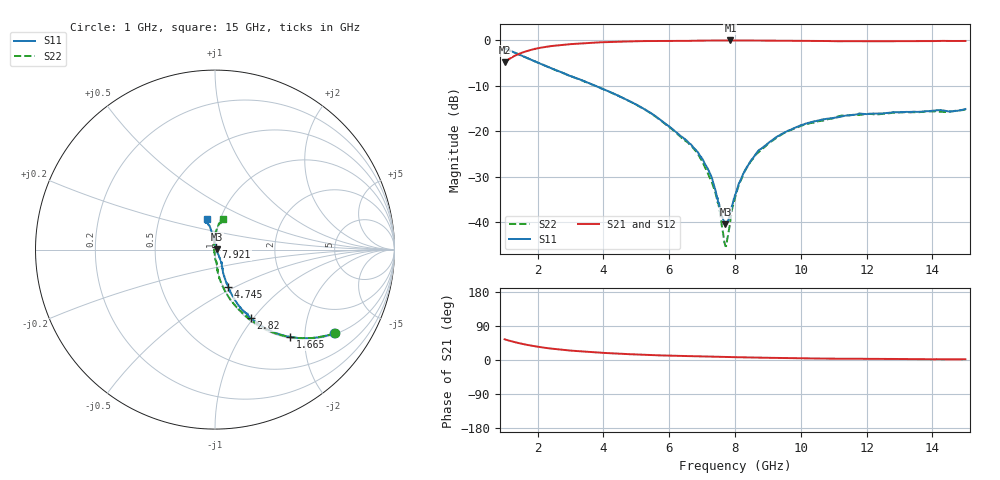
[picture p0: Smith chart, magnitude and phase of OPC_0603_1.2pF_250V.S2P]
! FILE NAME
! DATE 08/21/2012  10:43
! CORRECTED  DATA
# GHz  S  MA  R  50.00
!  FREQ  S11M  S11A  S21M  S21A  S12M  S12A  S22M  S22A
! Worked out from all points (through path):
!   1601 points, 1 GHz to 15 GHz, reference 50 ohm
!   highest |S21| = -0.06 dB at 7.86 GHz (marker M1); lowest = -4.8 dB at 1 GHz (marker M2)
!   group delay of S21, straight-line fit = 7.16 ps
!   lowest |S11| = -40.4 dB at 7.711 GHz (marker M3), VSWR 1.02, Z = 50.9 + j0.271 ohm
!   |S11| at or under -10 dB: 3.75 GHz to end of sweep
!   |S22| runs from -45.2 to -1.8 dB; largest |S21 - S12| = 0.0084
!   S11 on the Smith chart (normalised r, x): 1 GHz: 1.03, -2.83; 1.665 GHz: 1.03, -1.70; 2.82 GHz: 1.03, -0.97; 4.745 GHz: 1.05, -0.46; 7.921 GHz: 1.01, +0.03; 15 GHz: 0.87, +0.30
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1  0.8129 -35.0  0.5723 54.7  0.5721 54.5  0.813 -35.0
1.665  0.6423 -49.2  0.7569 40.3  0.7564 40.3  0.6422 -49.3
2.82  0.4303 -62.5  0.895 26.3  0.8946 26.4  0.4303 -63.9
3.33625  0.3644 -65.8  0.9239 22.6  0.9232 22.6  0.363 -68.0
4.745  0.2185 -70.6  0.9695 15.6  0.9692 15.5  0.2182 -77.6
5.6725  0.1385 -70.8  0.9834 12.4  0.983 12.3  0.1375 -82.8
6.62625  0.07298 -61.9  0.9839 10.2  0.9835 10.2  0.07131 -82.9
6.97625  0.05207 -59.7  0.9889 9.5  0.988 9.5  0.0485 -87.1
7.23875  0.03444 -56.0  0.9913 9.0  0.9909 9.0  0.03059 -91.4
7.39625  0.02308 -52.4  0.9925 8.6  0.992 8.6  0.02155 -96.1
7.62375  0.01111 -13.7  0.993 8.2  0.9923 8.2  0.008128 -126.1
7.71125  0.00954 16.2  0.993 8.0  0.9929 8.0  0.005548 -171.8
7.7725  0.01026 35.6  0.993 7.9  0.9927 7.9  0.006747 151.0
7.86  0.01298 60.2  0.9937 7.7  0.9928 7.7  0.01061 126.2
7.92125  0.01564 69.8  0.9933 7.6  0.9932 7.6  0.01445 113.9
8  0.01985 78.2  0.9935 7.5  0.9924 7.5  0.01858 110.4
8.28875  0.03616 92.3  0.9921 7.0  0.9917 7.0  0.03616 98.9
8.67375  0.05874 97.1  0.991 6.4  0.9906 6.4  0.05718 92.4
9.4875  0.09604 100.5  0.9883 5.3  0.988 5.2  0.09529 87.7
10.33625  0.1263 102.2  0.9837 4.2  0.983 4.1  0.1237 82.9
12.6725  0.1594 108.9  0.9719 2.8  0.9717 2.8  0.1575 77.7
15  0.1753 104.2  0.9814 2.0  0.9809 2.0  0.1732 75.6
